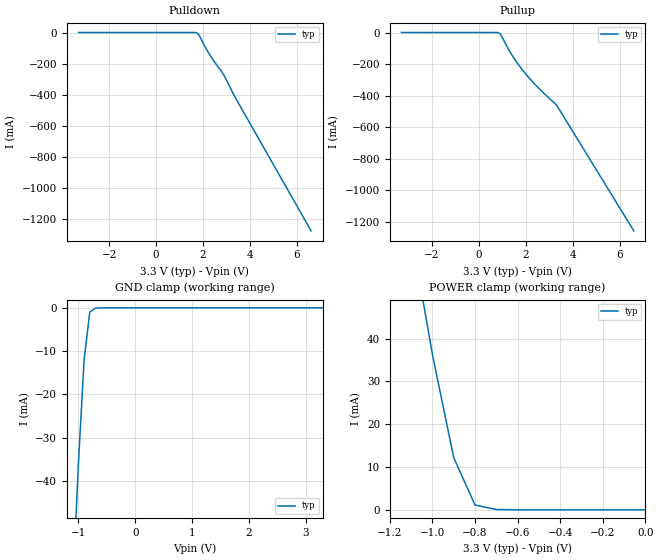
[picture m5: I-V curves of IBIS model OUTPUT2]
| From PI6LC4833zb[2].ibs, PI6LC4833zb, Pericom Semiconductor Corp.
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| Model  OUTPUT2 (PECL)
[Model]  OUTPUT2
Model_type  Output_ECL
Polarity Non-Inverting
Enable Active-High
Vmeas = 1.975V | Vmeas = ( VOH - VOL ) / 2 + VOL
Rref = 50.0
Cref = 0
Vref = 1.3V | Vref = vcc - 2V
C_comp   2pF   1.5pF   2.5pF
[Voltage Range]   3.30V   3.00V   3.60V
| Open source, no load
[POWER Clamp Reference]   3.30V   3.00V   3.60V
[Pullup Reference]   3.30V   3.00V   3.60V
[Pulldown Reference]   3.30V   3.00V   3.60V
[GND Clamp Reference]   0.00V   0.00V   0.00V
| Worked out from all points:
|   GND clamp passes 1 mA (typ) near -0.80 V on its own axis
|   POWER clamp passes 1 mA (typ) near -0.79 V on its own axis
[GND_clamp]
| voltage = voutput
| voltage   I(typ)   I(min)   I(max)
-3.3V     -1.04A     NA         NA
-1.1V     -64.4mA    NA         NA
-1V       -35.9mA    NA         NA
-900mV    -12mA      NA         NA
-800mV    -978uA     NA         NA
-700mV    -63.5uA    NA         NA
3.3V      13.2pA     NA         NA
[POWER_clamp]
| voltage = vcc - voutput
| voltage   I(typ)   I(min)   I(max)
-3.3V     783mA      NA         NA
-1.1V     64.9mA     NA         NA
-1V       36.3mA     NA         NA
-900mV    12.2mA     NA         NA
-800mV    1.13mA     NA         NA
-700mV    81.2uA     NA         NA
0V        13.2pA     NA         NA
[Pulldown]
| voltage = vcc - voutput
| voltage   I(typ)   I(min)   I(max)
-3.3V     0A         NA         NA
1.6V      -12.23uA   NA         NA
1.7V      -542.5uA   NA         NA
1.8V      -10.52mA   NA         NA
2.3V      -147.2mA   NA         NA
2.9V      -277.8mA   NA         NA
3.3V      -399.5mA   NA         NA
6.6V      -1.275A    NA         NA
[Pullup]
| voltage = vcc -voutput
| voltage   I(typ)   I(min)   I(max)
-3.3V     0A         NA         NA
700mV     -5.881uA   NA         NA
900mV     -6.916mA   NA         NA
1.4V      -140.7mA   NA         NA
1.9V      -245mA     NA         NA
2.5V      -345.4mA   NA         NA
3.3V      -457.6mA   NA         NA
6.6V      -1.257A    NA         NA
[Ramp]
| variable typ min max
dV/dt_r 450m/444.42p  NA NA
dV/dt_f 450m/275.22p   NA NA
R_load = 50.00
